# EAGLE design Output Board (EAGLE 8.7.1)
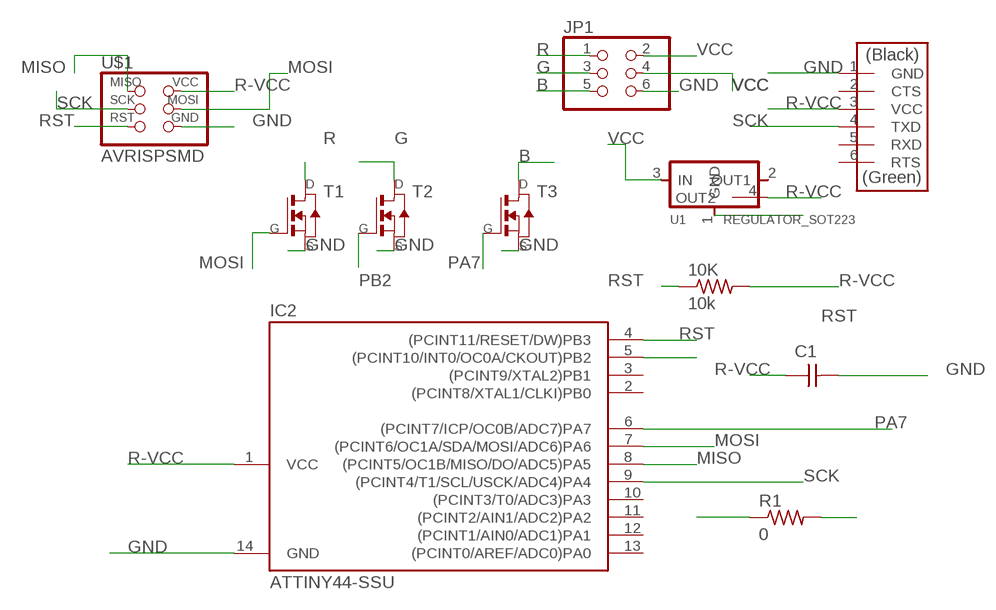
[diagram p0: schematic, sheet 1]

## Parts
10K  10k  RES-US1206  [R1206]
C1  CAP-UNPOLARIZED  [C1206]
IC2  ATTINY44-SSU  [SOIC14]
JP1  PINHD-2X3-SMD  [2X03SMD]
R1  0  RES-US1206  [R1206]
T1  NMOSFETSOT23  [SOT-23]
T2  NMOSFETSOT23  [SOT-23]
T3  NMOSFETSOT23  [SOT-23]
U1  REGULATOR_SOT223  [SOT223]
U$1  AVRISPSMD  [2X03SMD]
U$2  FTDI-SMD-HEADER  [1X06SMD]

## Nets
B: JP1.5 T3.1(D)
G: JP1.3 T2.1(D)
GND: C1.2 IC2.14(GND) JP1.6 R1.1 R1.2 T1.2(S) T2.2(S) T3.2(S) U1.1(GND) U$1.6(GND) U$2.1(GND)
MISO: IC2.8((PCINT5/OC1B/MISO/DO/ADC5)PA5) U$1.1(MISO)
MOSI: IC2.7((PCINT6/OC1A/SDA/MOSI/ADC6)PA6) T1.3(G) U$1.4(MOSI)
PA7: IC2.6((PCINT7/ICP/OC0B/ADC7)PA7) T3.3(G)
PB2: IC2.5((PCINT10/INT0/OC0A/CKOUT)PB2) T2.3(G)
R: JP1.1 T1.1(D)
R-VCC: 10K.2 C1.1 IC2.1(VCC) U1.4(OUT2) U$1.2(VCC) U$2.3(VCC)
RST: 10K.1 IC2.4((PCINT11/RESET/DW)PB3) U$1.5(RST)
SCK: IC2.9((PCINT4/T1/SCL/USCK/ADC4)PA4) U$1.3(SCK) U$2.4(TXD)
VCC: JP1.2 JP1.4 U1.3(IN)
Unconnected: IC2.2((PCINT8/XTAL1/CLKI)PB0) IC2.3((PCINT9/XTAL2)PB1) IC2.10((PCINT3/T0/ADC3)PA3) IC2.11((PCINT2/AIN1/ADC2)PA2) IC2.12((PCINT1/AIN0/ADC1)PA1) IC2.13((PCINT0/AREF/ADC0)PA0) U1.2(OUT1) U$2.2(CTS) U$2.5(RXD) U$2.6(RTS)

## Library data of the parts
10K R1 = fab:RES-US: Resistor (US Symbol)
C1 = fab:CAP-UNPOLARIZED
IC2 = fab:ATTINY44
JP1 = fab:PINHD-2X3-SMD: PIN HEADER
T1-T3 = fab:NMOSFET: MOS FET
U1 = fab:REGULATOR_SOT223
U$1 = fab:AVRISP
U$2 = fab:FTDI-SMD-HEADER

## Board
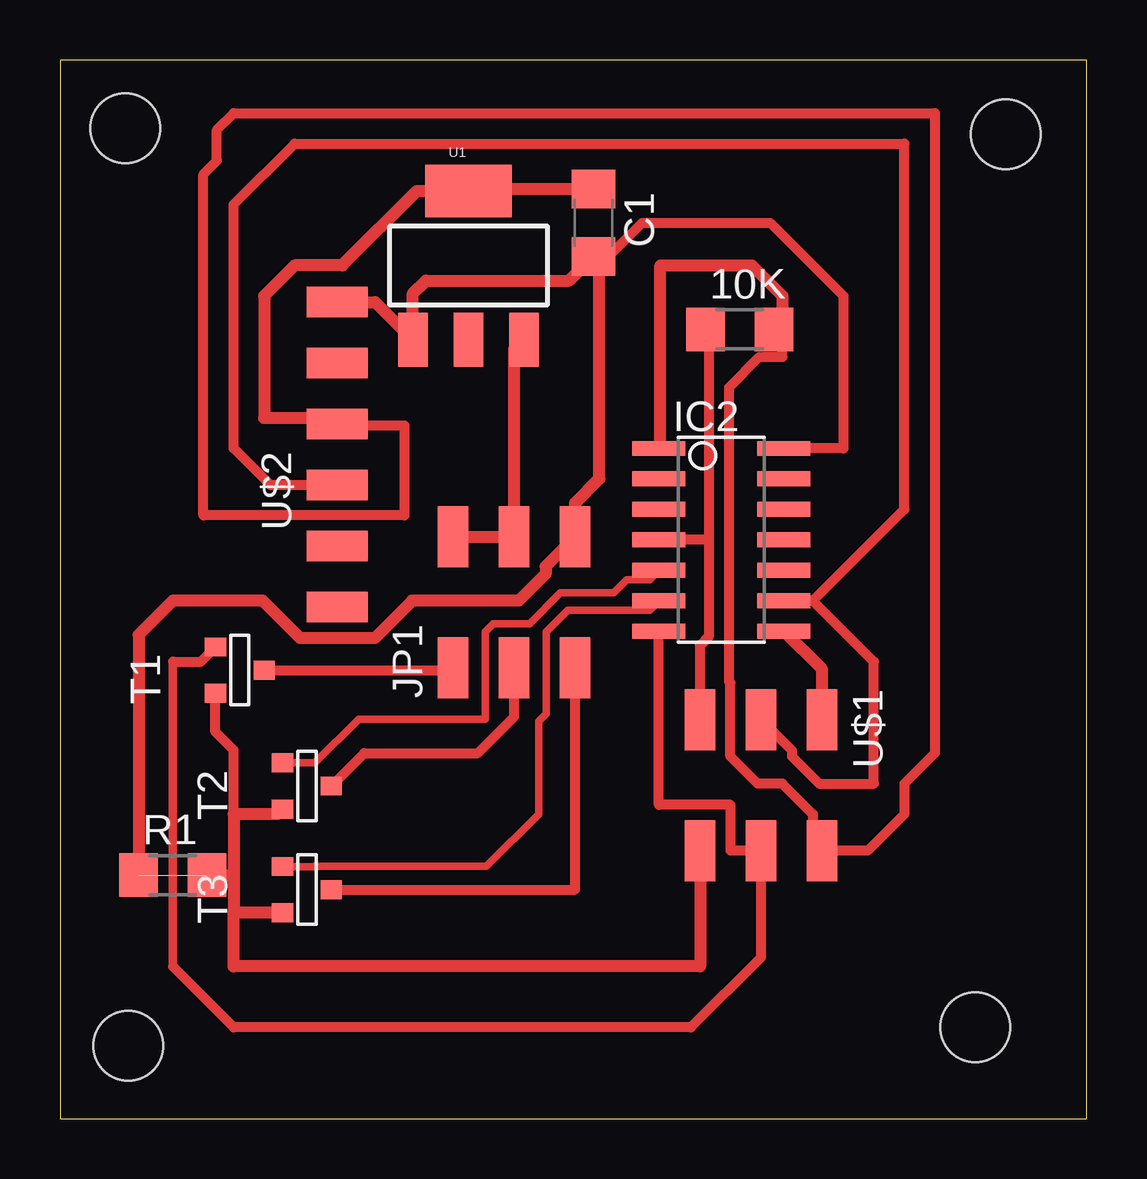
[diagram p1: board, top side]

Size 42.78 x 44.12 mm. Coordinates in mm from the lower left corner, seen from the top.
Outline: 0,0 42.78,0 42.78,44.12 0,44.12 0,0
Copper layers (1*16): Top 0.035mm / dielectric 1.5mm / Bottom 0.035mm
Design rules "fabmodule (2)": minimum track width 10mil, minimum drill 0.4mm, track to track 0.42mm, track to pad 0.42mm, pad to pad 0.42mm, via to via 0.42mm, smd to smd 0.42mm, copper to edge 40mil, drill to drill 0.8mm, minimum pad ring 10mil, minimum via ring 8mil, stop-mask expansion 4mil, vias tented up to drill 0mil, thermal gap 10mil
Holes 2.9 mm at 2.73,41.28 39.41,41.03 2.85,3.05 38.14,3.81

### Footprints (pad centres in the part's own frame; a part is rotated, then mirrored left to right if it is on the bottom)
R1206 = smd 1.6 x 1.803: 1 -1.422,0; 2 1.422,0
C1206 = smd 1.6 x 1.8: 1 -1.4,0; 2 1.4,0
SOIC14 = smd 0.61 x 2.21: 1 -3.81,-2.603; 2 -2.54,-2.603; 3 -1.27,-2.603; 4 0,-2.603; 5 1.27,-2.603; 6 2.54,-2.603; 7 3.81,-2.603; 8 3.81,2.603; 9 2.54,2.603; 10 1.27,2.603; 11 0,2.603; 12 -1.27,2.603; 13 -2.54,2.603; 14 -3.81,2.603
2X03SMD = smd 2.54 x 1.27: 1 -2.54,2.54; 2 2.92,2.54; 3 -2.54,0; 4 2.92,0; 5 -2.54,-2.54; 6 2.92,-2.54
SOT-23 = smd 0.787 x 0.889: 1 0.025,-1.016; 2 -0.94,1.016; 3 0.991,1.016
SOT223 = smd 1.219 x 2.235: 1 -2.311,-3.099; 2 0,-3.099; 3 2.311,-3.099 | smd 3.6 x 2.2: 4 0,3.099
1X06SMD = smd 2.54 x 1.27: 1 0,6.35; 2 0,3.81; 3 0,1.27; 4 0,-1.27; 5 0,-3.81; 6 0,-6.35

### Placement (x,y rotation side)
10K  28.32,32.89 0 top
C1  22.23,37.34 270 top
IC2  27.56,24.13 270 top
JP1  18.92,21.34 90 top
R1  4.7,10.16 0 top
T1  7.49,18.67 90 top
T2  10.29,13.84 90 top
T3  10.29,9.53 90 top
U1  17.02,35.56 0 top
U$1  29.21,14.1 270 top
U$2  11.56,27.69 0 top

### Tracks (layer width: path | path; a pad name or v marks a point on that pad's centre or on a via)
B
  Top 0.406: T3.1 21.46,9.55 JP1.5
G
  Top 0.406: T2.1 12.67,15.24 17.4,15.24 18.92,16.76 JP1.3
GND  (1 unrouted)
  Top 0.406: T2.2 9.07,12.7 | 7.24,12.7 7.24,15.37 6.48,16.13 T1.2 | C1.2 22.86,35.94 24.26,37.34 29.59,37.34 32.64,34.29 32.64,27.94 IC2.14
  Top 0.508: T3.2 7.24,8.58 | 7.24,10.16 7.24,12.7 9.07,12.7 | 7.24,10.16 7.24,8.58 | U$1.6 26.67,6.35 7.24,6.35 7.24,8.58 | R1.2 7.24,10.16 | R1.1 3.28,20.17 4.7,21.59 8.45,21.59 10.01,20.03 13.11,20.03 14.67,21.59 19.12,21.59 20.23,22.71 20.23,23.02 JP1.6 21.46,25.65 22.48,26.67 22.48,35.68 C1.2 21.21,34.93 15.24,34.93 14.71,34.39 U1.1 13.13,34.04 U$2.1
MISO
  Top 0.508: U$1.1 31.75,18.73 IC2.8
MOSI
  Top 0.356: 4.7,6.35 4.7,19.05
  Top 0.406: IC2.7 24.96,13.08 27.94,13.08 27.94,11.18 U$1.4 29.21,6.73 26.29,3.81 7.24,3.81 4.7,6.35 | 4.7,19.05 5.87,19.05 T1.3
PA7
  Top 0.305: IC2.6 24.56,21.2 21.15,21.2 20.26,20.3 20.26,16.89 19.94,16.57 19.94,12.7 17.76,10.52 10.62,10.52 | 10.62,10.52 | 10.62,10.52 T3.3
PB2
  Top 0.305: IC2.5 24.56,22.47 23.61,22.47 23.07,21.92 20.85,21.92 19.57,20.64 18.05,20.64 17.72,20.3 17.72,16.65 12.44,16.65 10.62,14.83 T2.3
R
  Top 0.406: T1.1 16.28,18.69 JP1.1
R-VCC
  Top 0.406: 10K.2 30.1,32.89 30.1,31.75 29.15,31.75 27.88,30.48 27.88,18.22 27.93,18.16 27.93,15.11 29.07,13.97 30.1,13.97 31.37,12.7 31.37,11.56 U$1.2 33.66,11.18 35.18,12.7 35.18,13.97 36.45,15.24 36.45,41.91 7.24,41.91 6.54,41.21 6.54,39.92 5.97,39.36 5.97,25.15 14.35,25.15 14.35,28.89 11.56,28.89 U$2.3
  Top 0.508: IC2.1 25.02,28 25.02,35.56 28.83,35.56 30.1,34.29 30.1,32.89 | 22.15,38.66 C1.1 17.1,38.74 U1.4 14.87,38.66 11.77,35.56 9.78,35.56 8.51,34.29 8.51,29.21 11.24,29.21 11.56,28.89
RST
  Top 0.406: U$1.5 26.67,19.74 27.05,20.12 27.05,24.13 | 27.05,24.13 IC2.4 | 27.05,24.13 27.05,32.74 10K.1
SCK
  Top 0.406: 31.37,21.59 35.18,25.4 35.18,40.64 9.78,40.64 7.24,38.1 7.24,27.94 8.76,26.42 U$2.4 | 31.37,21.59 IC2.9 | U$1.3 30.49,15.35 30.49,15.11 31.63,13.97 33.91,13.97 33.91,19.05 31.37,21.59
VCC
  Top 0.406: JP1.4 18.92,24.99
  Top 0.508: JP1.2 JP1.4 | JP1.4 18.84,24.34 | JP1.4 18.92,32.05 U1.3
